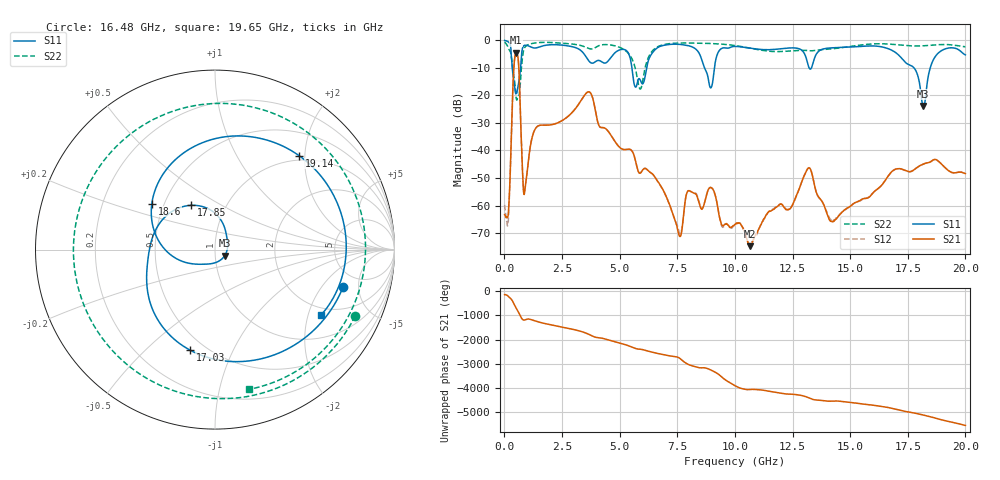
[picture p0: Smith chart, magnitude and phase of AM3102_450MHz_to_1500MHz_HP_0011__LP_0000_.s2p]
!Agilent Technologies,E8364B,MY43040894,A.07.50.67
!Agilent E8364B: A.07.50.67
!Date: Thursday, January 11, 2018 05:29:49
!Correction: S11(Full 2 Port(1,2))
!S21(Full 2 Port(1,2))
!S12(Full 2 Port(1,2))
!S22(Full 2 Port(1,2))
!S2P File: Measurements: S11, S21, S12, S22:
# Hz S  dB  R 50
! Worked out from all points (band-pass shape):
!   1601 points, 10 MHz to 20 GHz, reference 50 ohm
!   highest |S21| = -4.53 dB at 509.8 MHz (marker M1); lowest = -74.7 dB at 10.64 GHz (marker M2)
!   |S21| within 3 dB of the highest: 433.7 MHz to 606.3 MHz (172.6 MHz wide, 33.2 % of centre)
!   lowest |S11| = -23.9 dB at 18.18 GHz (marker M3), VSWR 1.14, Z = 55.6 - j3.74 ohm
!   |S11| at or under -10 dB: 5.531 GHz to 6.172 GHz (640.4 MHz wide, 10.9 % of centre); 8.684 GHz to 9.111 GHz (427.1 MHz wide, 4.8 % of centre); 17.77 GHz to 18.47 GHz (703.9 MHz wide, 3.88 % of centre)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
!   |S22| runs from -21.7 to -0.6 dB; largest |S21 - S12| = 0.0022
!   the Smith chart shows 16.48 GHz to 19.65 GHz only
!   S11 on the Smith chart (normalised r, x): 16.48 GHz: 3.57, -3.32; 17.03 GHz: 0.41, -0.69; 17.85 GHz: 0.68, +0.37; 18.6 GHz: 0.43, +0.27; 19.14 GHz: 0.91, +1.88; 19.65 GHz: 1.73, -2.43
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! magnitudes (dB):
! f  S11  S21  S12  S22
! 10 MHz  0.0  -63.3  -59.7  -0.6
! 172.4 MHz  -0.6  -62.8  -65.4  -2.8
! 509.8 MHz  -18.6  -4.5  -4.5  -20.8
! 884.6 MHz  -1.8  -54.7  -54.5  -2.5
! 3.346 GHz  -3.9  -21.6  -21.6  -2.0
! 5.895 GHz  -14.4  -48.2  -48.2  -17.7
! 6.682 GHz  -2.5  -51.6  -51.6  -2.2
! 7.606 GHz  -1.5  -71.2  -70.0  -1.0
! 8.018 GHz  -2.0  -54.6  -54.7  -1.0
! 10.01 GHz  -2.2  -66.8  -66.9  -1.9
! 10.64 GHz  -2.8  -74.7  -74.1  -2.8
! 13.34 GHz  -9.6  -48.3  -48.3  -3.8
! 14.22 GHz  -2.7  -65.8  -65.4  -3.1
! 16.48 GHz  -2.6  -51.4  -51.4  -1.3
! 16.68 GHz  -3.1  -49.0  -49.0  -1.4
! 17.03 GHz  -4.8  -46.7  -46.7  -1.6
! 17.85 GHz  -11.0  -46.5  -46.5  -2.1
! 18.18 GHz  -23.9  -44.9  -44.9  -2.0
! 18.6 GHz  -7.2  -43.5  -43.5  -1.7
! 19.14 GHz  -3.1  -46.4  -46.4  -1.5
! 19.65 GHz  -3.2  -47.9  -48.0  -1.9
! 20 GHz  -5.3  -48.4  -48.4  -2.3
